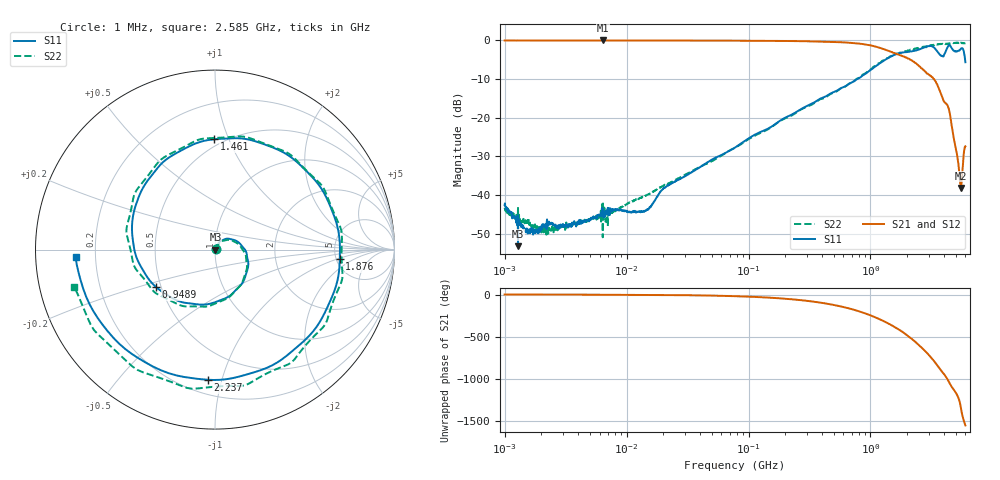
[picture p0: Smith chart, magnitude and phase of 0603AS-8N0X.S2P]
!s-Parameter Generated by FASTRON Sdn. Bhd.
!FASTRON P/N : 0603AS-8N0X
!Keysight Technologies: E5071C_MY46733604_B.14.02
!Date: Mon Dec 04 09:47:02 2023
!Version  :Rev01  Mon Dec 04 09:47:02 2023
!Data & Calibration Information:
!Freq  S11:SOLT2(ON)  S21:SOLT2(ON)  S12:SOLT2(ON)  S22:SOLT2(ON)
!PortZ  Port1:50+j0  Port2:50+j0
!When reading reference impedance value at option line is always used.
! Remarks : This data is being provided solely for informational purposes.
# Hz S dB R 50
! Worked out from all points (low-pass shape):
!   1601 points, 1 MHz to 6 GHz, reference 50 ohm
!   highest |S21| = -0.03 dB at 6.378 MHz (marker M1); lowest = -38.2 dB at 5.496 GHz (marker M2)
!   |S21| within 3 dB of the highest: start of sweep to 1.5 GHz
!   lowest |S11| = -53.2 dB at 1.288 MHz (marker M3), VSWR 1.00, Z = 50.2 + j0.0541 ohm
!   |S11| at or under -10 dB: start of sweep to 779 MHz
!   |S22| runs from -50.9 to -0.6 dB; largest |S21 - S12| = 0.0027
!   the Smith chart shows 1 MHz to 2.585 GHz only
!   S11 on the Smith chart (normalised r, x): 1 MHz: 1.01, +0.01; 948.9 MHz: 0.47, -0.23; 1.461 GHz: 0.45, +0.89; 1.876 GHz: 5.37, -1.11; 2.237 GHz: 0.29, -0.90; 2.585 GHz: 0.12, -0.03
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1000000  -42.63 25.0  -0.04 -0.1  -0.04 -0.2  -43.29 22.9
1287650  -53.24 14.3  -0.04 -0.2  -0.03 -0.2  -43.06 6.4
4277066  -47.36 46.8  -0.05 -1.1  -0.04 -1.1  -47.15 46.5
6378092  -45.31 61.3  -0.03 -1.7  -0.04 -1.7  -50.94 55.4
1.823719e7  -39.92 64.4  -0.05 -4.7  -0.05 -4.6  -38.28 59.7
7.757876e7  -27.73 61.5  -0.08 -19.5  -0.09 -19.4  -27.76 58.2
3.307917e8  -16.37 7.0  -0.26 -81.7  -0.26 -81.7  -16.63 3.7
6.68109e8  -11.25 -75.0  -0.61 -164.7  -0.61 -164.7  -11.19 -73.2
9.488551e8  -8.20 -147.4  -1.16 125.7  -1.16 125.7  -7.97 -140.3
1.414819e9  -4.45 101.2  -2.75 13.3  -2.75 13.4  -4.41 104.7
1.461095e9  -4.22 90.3  -2.93 3.0  -2.93 3.0  -4.13 95.0
1.875526e9  -3.13 -4.4  -4.16 -93.4  -4.17 -93.3  -3.03 -0.8
2.23694e9  -2.78 -93.2  -5.46 -178.4  -5.45 -178.3  -2.29 -81.3
2.584893e9  -2.18 -176.8  -7.08 100.1  -7.04 100.3  -1.82 -165.1
3.083002e9  -1.47 74.0  -9.16 -12.1  -9.11 -12.3  -1.29 81.1
3.482718e9  -2.62 -24.6  -11.17 -108.1  -11.15 -108.5  -1.01 -7.3
3.867453e9  -4.06 -122.3  -14.65 164.6  -14.68 164.3  -0.89 -97.8
4.231938e9  -2.05 163.3  -16.64 87.2  -16.67 86.9  -0.89 176.4
4.628987e9  -1.99 81.3  -22.02 -12.2  -22.06 -12.3  -0.70 89.6
5.048685e9  -2.93 14.5  -28.52 -91.4  -28.55 -91.4  -0.60 -0.7
5.496363e9  -2.18 -78.6  -38.17 107.5  -38.20 107.5  -0.62 -97.3
6e9  -5.66 111.1  -27.44 -111.1  -27.43 -111.0  -0.72 161.4
